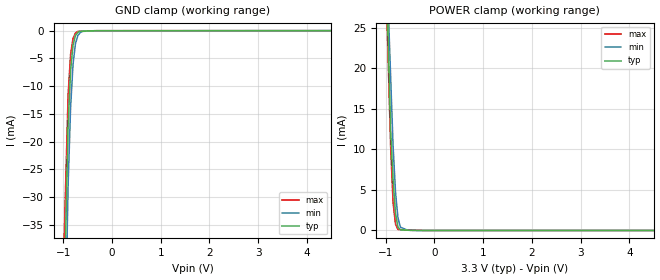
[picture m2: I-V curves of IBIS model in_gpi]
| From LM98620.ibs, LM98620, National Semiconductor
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[Model] in_gpi
Model_type Input
Vinl = 800.000mV
Vinh = 2.00000V
C_comp 783.000fF 740.000fF 814.000fF
| variable typ   min   max
[Voltage Range] 3.30000V 3.00000V 3.60000V
[POWER Clamp Reference] 3.30000V 3.00000V 3.60000V
[GND Clamp Reference] 0.00000V 0.00000V 0.00000V
[Temperature Range]   25   70   0
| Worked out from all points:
|   GND clamp passes 1 mA (typ) near -0.75 V on its own axis
|   POWER clamp passes 1 mA (typ) near -0.77 V on its own axis
[GND Clamp]
-3.3V     -943.1mA   -1.096A    -775.4mA
-900mV    -16.97mA   -27.68mA   -11.4mA
-850mV    -7.232mA   -13.94mA   -4.313mA
-800mV    -2.625mA   -6.091mA   -1.394mA
-750mV    -867.2uA   -2.342mA   -420.3uA
-700mV    -285.3uA   -862.3uA   -127.1uA
-650mV    -103.5uA   -345.4uA   -109.3uA
-600mV    -88.99uA   -124.2uA   -91.56uA
-350mV    -16.46uA   -32.42uA   -2.684uA
-325mV    -9.202uA   -23.24uA   -2.65uA
-300mV    -9.138uA   -14.07uA   -2.617uA
6.6V      8.702uA    16.17uA    6.551uA
[POWER Clamp]
-3.3V     548.7mA    429.3mA    810.1mA
-1.05V    45.83mA    44.61mA    41.38mA
-900mV    12.31mA    18.96mA    10.36mA
-850mV    6.229mA    10.41mA    3.436mA
-800mV    2.078mA    4.727mA    791.6uA
-750mV    426.5uA    1.567mA    118uA
-700mV    68.53uA    408.4uA    106.8uA
-550mV    39.16uA    33.35uA    73.07uA
-450mV    19.58uA    0A         50.59uA
6.6V      0A         0A         0A
